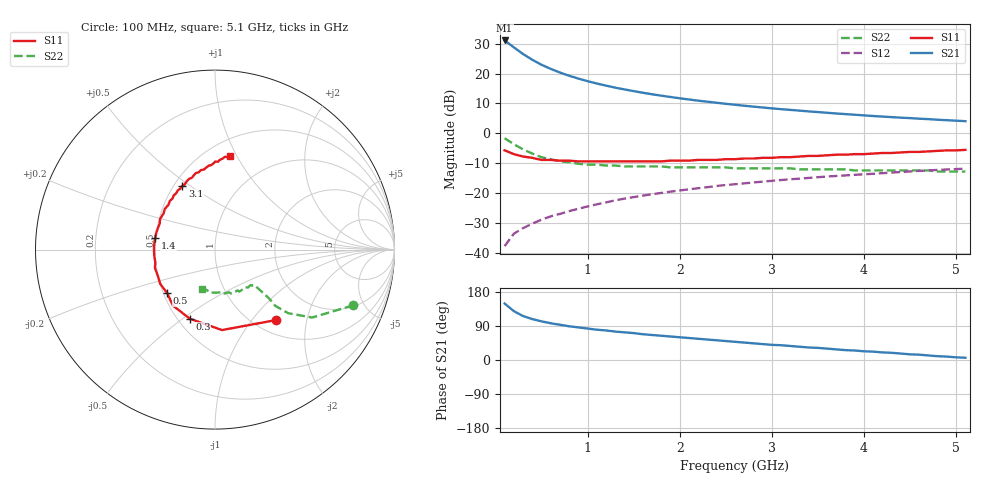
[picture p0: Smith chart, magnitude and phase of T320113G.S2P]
!AT-32011
!S and NOISE PARAMETERS at Vce=2.7 V  Ic=20mA.  LAST UPDATED 01-05-95
# ghz s ma r 50
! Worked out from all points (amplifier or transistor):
!   51 points, 100 MHz to 5.1 GHz, reference 50 ohm
!   highest |S21| = 31.1 dB at 100 MHz (marker M1)
!   |S21| within 3 dB of that: start of sweep to 231.5 MHz
!   unconditionally stable (mu >= 1): 893.5 MHz to 4.675 GHz
!   at 900 MHz: K = 1.00, MAG = 21.5 dB, |S12| = -25.2 dB
!   at 2.6 GHz: K = 1.08, MAG = 11.6 dB, |S12| = -17.0 dB
!   at 5.1 GHz: K = 0.98, MSG = 7.9 dB, |S12| = -11.8 dB
!   lowest NFmin = 1.39 dB at 500 MHz
!   S11 on the Smith chart (normalised r, x): 100 MHz: 1.24, -1.33; 300 MHz: 0.57, -0.53; 500 MHz: 0.52, -0.29; 1.4 GHz: 0.50, +0.07; 3.1 GHz: 0.55, +0.47; 5.1 GHz: 0.64, +0.94
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0.1  0.52 -49.0  35.79 149.0  0.013 72.0  0.83 -22.0
0.2  0.45 -85.0  27.47 129.0  0.021 63.0  0.66 -35.0
0.3  0.41 -110.0  21.25 116.0  0.026 61.0  0.54 -41.0
0.4  0.39 -127.0  17.01 108.0  0.031 61.0  0.46 -43.0
0.5  0.36 -138.0  14.06 102.0  0.036 62.0  0.4 -42.0
0.6  0.36 -148.0  11.98 97.0  0.041 63.0  0.37 -42.0
0.7  0.35 -156.0  10.41 93.0  0.045 63.0  0.34 -42.0
0.8  0.35 -163.0  9.2 89.0  0.05 64.0  0.33 -42.0
0.9  0.34 -168.0  8.25 86.0  0.055 64.0  0.31 -42.0
1  0.34 -174.0  7.47 83.0  0.06 64.0  0.3 -42.0
1.1  0.34 -178.0  6.82 80.0  0.065 64.0  0.3 -42.0
1.2  0.34 178.0  6.29 78.0  0.07 64.0  0.29 -43.0
1.4  0.34 169.0  5.43 73.0  0.081 63.0  0.28 -45.0
1.6  0.34 162.0  4.78 68.0  0.091 62.0  0.28 -47.0
1.8  0.34 155.0  4.27 64.0  0.101 61.0  0.28 -49.0
2.2  0.36 141.0  3.52 56.0  0.121 58.0  0.27 -55.0
2.6  0.37 130.0  3.01 48.0  0.141 55.0  0.26 -61.0
3.1  0.4 117.0  2.54 39.0  0.166 51.0  0.26 -69.0
3.5  0.42 108.0  2.27 32.0  0.185 47.0  0.25 -75.0
3.8  0.44 102.0  2.1 26.0  0.198 44.0  0.25 -80.0
4.3  0.47 93.0  1.87 19.0  0.221 40.0  0.24 -89.0
5.1  0.53 81.0  1.6 6.0  0.257 31.0  0.23 -108.0
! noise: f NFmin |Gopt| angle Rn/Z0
0.5  1.39  0.15  65  0.16
0.9  1.51  0.14  105  0.13
1.8  1.78  0.28  -164  0.12
2.4  1.96  0.4  -142  0.13
